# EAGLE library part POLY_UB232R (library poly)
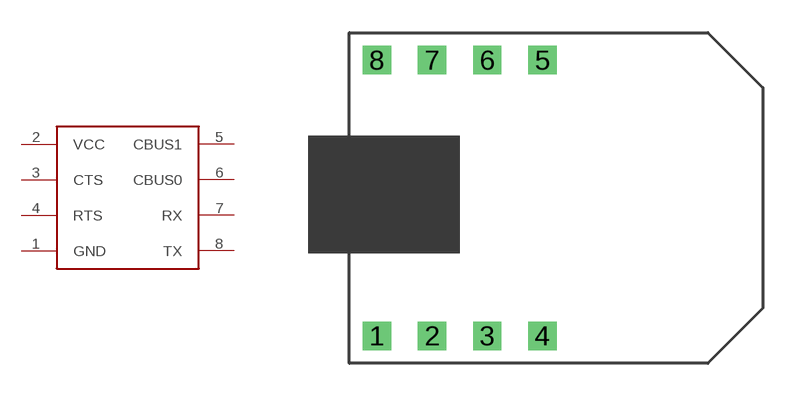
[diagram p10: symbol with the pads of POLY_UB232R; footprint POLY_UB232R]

Designator prefix -

## POLY_UB232R  [POLY_UB232R]
1  GND  pwr
2  VCC  sup
3  CTS
4  RTS
5  CBUS1
6  CBUS0
7  RX  in
8  TX  out

## Footprint POLY_UB232R (pad centres in mm)
drill 0.8 square: 1 -7.62,-6.35; 2 -5.08,-6.35; 3 -2.54,-6.35; 4 0,-6.35; 5 0,6.35; 6 -2.54,6.35; 7 -5.08,6.35; 8 -7.62,6.35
